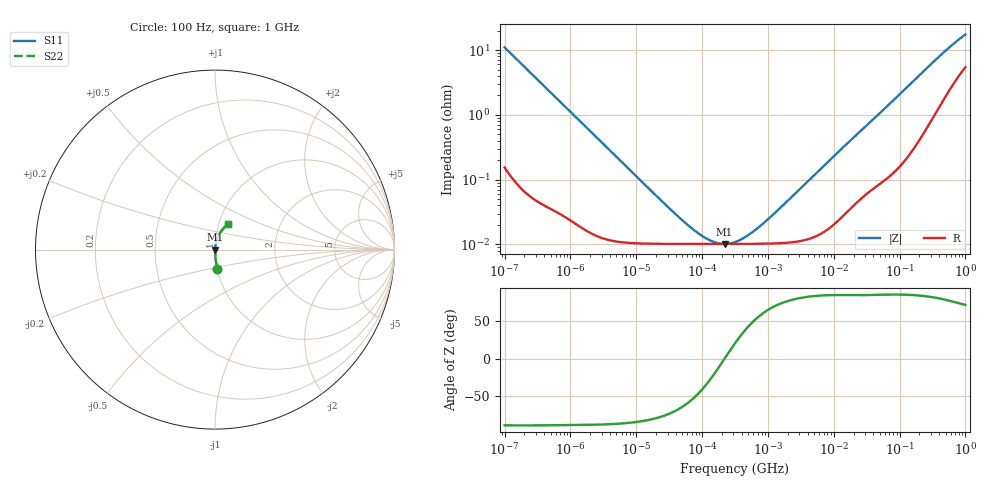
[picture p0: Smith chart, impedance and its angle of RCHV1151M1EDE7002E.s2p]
! RCHV1151M1EDE7002E  S-PARAMETER MODEL  (AEC-Q200 qualified)
! Model Generated by ELNA Corporation (http://www.ty-top.com)
! Version 1.0
! ELNA Control No.240229
! Copyright (c) 2024 ELNA CO.,LTD. All Rights Reserved.
! Products Name : CONDUCTIVE POLYMER HYBRID ALUMINUM ELECTROLYTIC CAPACITORS
! Characteristics :
!  Capacitance  :  150uF  ,  Rated voltage  :  16V
!  Operating Temp. Range  :  -55 to +105 degC  ,  Endurance  :  10000hr at 105 degC
!  Dimension D  :  6.3mm  ,  Dimension L  :  7.7mm
! Frequency Range : 100Hz - 1GHz
! External Node Assignments :
!  1  o---| |---o  2
# MHz S RI R 50
!Freq[MHz].  S11 Real  S11 Imag  S21 Real  S21 Imag  S12 Real  S12 Imag  S22 Real  S22 Imag
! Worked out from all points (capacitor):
!   401 points, 100 Hz to 1 GHz, reference 50 ohm
!   read as one part in series: C = 145 uF near 108 Hz
!   lowest |Z| = 10.2 mohm at 220 kHz (marker M1)
!   series resonance near 219.8 kHz, so ESL is about 3.6 nH
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0.0001  0.0134 -0.1083  0.9866 0.1083  0.9866 0.1083  0.0134 -0.1083
0.000113  0.0107 -0.0963  0.9893 0.0963  0.9893 0.0963  0.0107 -0.0963
0.000309  0.00173 -0.0356  0.9983 0.0356  0.9983 0.0356  0.00173 -0.0356
0.001488  0.000236 -0.00751  0.9998 0.00751  0.9998 0.00751  0.000236 -0.00751
0.022131  0.000102 -0.000503  0.9999 0.000503  0.9999 0.000503  0.000102 -0.000503
0.051582  0.000102 -0.000206  0.9999 0.000206  0.9999 0.000206  0.000102 -0.000206
0.090678  0.000102 -0.000103  0.9999 0.000103  0.9999 0.000103  0.000102 -0.000103
0.115478  0.000102 -7.05e-05  0.9999 7.05e-05  0.9999 7.05e-05  0.000102 -7.05e-05
0.147062  0.000102 -4.22e-05  0.9999 4.22e-05  0.9999 4.22e-05  0.000102 -4.22e-05
0.179887  0.000102 -2.06e-05  0.9999 2.06e-05  0.9999 2.06e-05  0.000102 -2.06e-05
0.220039  0.000102 1.19e-07  0.9999 -1.19e-07  0.9999 -1.19e-07  0.000102 1.19e-07
0.316228  0.000102 3.8e-05  0.9999 -3.8e-05  0.9999 -3.8e-05  0.000102 3.8e-05
0.473151  0.000102 8.63e-05  0.9999 -8.63e-05  0.9999 -8.63e-05  0.000102 8.63e-05
0.767361  0.000102 0.000164  0.9999 -0.000164  0.9999 -0.000164  0.000102 0.000164
1.462177  0.000104 0.000332  0.9999 -0.000332  0.9999 -0.000332  0.000104 0.000332
4.704354  0.000127 0.00109  0.9999 -0.00109  0.9999 -0.00109  0.000127 0.00109
13.4122  0.000275 0.00304  0.9997 -0.00304  0.9997 -0.00304  0.000275 0.00304
69.9842  0.00133 0.0146  0.9987 -0.0146  0.9987 -0.0146  0.00133 0.0146
184.0772  0.00496 0.0373  0.995 -0.0373  0.995 -0.0373  0.00496 0.0373
412.0975  0.0199 0.0781  0.9801 -0.0781  0.9801 -0.0781  0.0199 0.0781
695.825  0.046 0.1168  0.954 -0.1168  0.954 -0.1168  0.046 0.1168
1000  0.0744 0.1451  0.9256 -0.1451  0.9256 -0.1451  0.0744 0.1451
